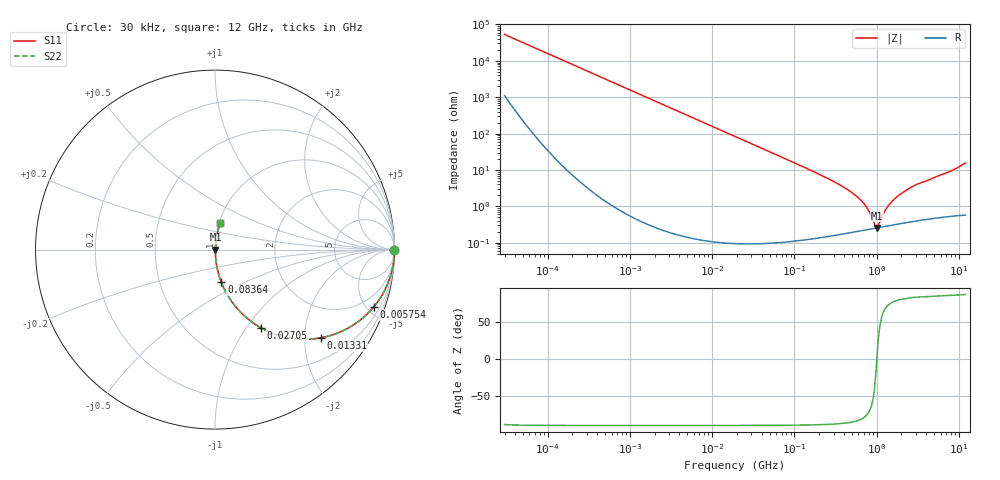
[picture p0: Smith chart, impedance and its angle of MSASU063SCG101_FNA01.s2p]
! MSASU063SCG101_FNA01  S-PARAMETER MODEL  ( General Type )
! Model Generated by TAIYO YUDEN Corporation (http://www.ty-top.com)
! Version 1.0
! TAIYO YUDEN Control No. 130520
! Copyright(c) 2013 TAIYO YUDEN CO.,LTD. All Rights Reserved.
! Product Description (link to TY-COMPAS)
! https://ds.yuden.co.jp/TYCOMPAS/or/detail?pn=MSASU063SCG101JFNA01&u=M
! Products Name : Multilayer Ceramic Capacitors
! Characteristics :
!  Capacitance : 100 pF , Rated Voltage : 50V , TCC : CG / C0G
!  Case Size : 0.6 x 0.3 / 0.024 x 0.012 [mm/inch] , Thickness : 0.3 / 0.012 [mm/inch]
!  (Conditions: Temperature = 25 degC , DC Bias Current/Voltage = 0A / 0V)
! External Node Assignments :
!  1  o---| |---o  2
! GND o---------o GND
! Frequency Range : 0.03MHz  -  12000MHz  [ 401 STEP ]
# MHz S RI R 50
! Freq[MHz].  S11 Real  S11 Imag  S21 Real  S21 Imag  S12 Real  S12 Imag  S22 Real  S22 Imag
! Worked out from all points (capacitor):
!   401 points, 30 kHz to 12 GHz, reference 50 ohm
!   read as one part in series: C = 99.9 pF near 32 kHz
!   lowest |Z| = 256 mohm at 1.002 GHz (marker M1)
!   series resonance near 1.004 GHz, so ESL is about 250 pH
!   S11 on the Smith chart (normalised r, x): 30 kHz: open; 5.754 MHz: 1.00, -5.54; 13.31 MHz: 1.00, -2.39; 27.05 MHz: 1.00, -1.18; 83.64 MHz: 1.00, -0.38; 12 GHz: 1.01, +0.31
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0.03  1 -0.00188  4.27e-05 0.00188  4.27e-05 0.00188  1 -0.00188
0.260295  0.9997 -0.0163  0.000279 0.0163  0.000279 0.0163  0.9997 -0.0163
2.258455  0.9802 -0.139  0.0198 0.139  0.0198 0.139  0.9802 -0.139
5.753879  0.8844 -0.3195  0.1156 0.3195  0.1156 0.3195  0.8844 -0.3195
13.30744  0.5887 -0.4917  0.4113 0.4917  0.4113 0.4917  0.5887 -0.4917
18.97367  0.4133 -0.4919  0.5867 0.4919  0.5867 0.4919  0.4133 -0.4919
27.05253  0.2574 -0.4364  0.7426 0.4364  0.7426 0.4364  0.2574 -0.4364
45.32004  0.1102 -0.3118  0.8898 0.3118  0.8898 0.3118  0.1102 -0.3118
83.63502  0.0355 -0.1822  0.9645 0.1822  0.9645 0.1822  0.0355 -0.1822
164.6252  0.01 -0.0931  0.99 0.0931  0.99 0.0931  0.01 -0.0931
356.9603  0.00319 -0.0388  0.9968 0.0388  0.9968 0.0388  0.00319 -0.0388
560.6502  0.00239 -0.0195  0.9976 0.0195  0.9976 0.0195  0.00239 -0.0195
749.4426  0.00235 -0.00942  0.9976 0.00942  0.9976 0.00942  0.00235 -0.00942
939.2353  0.00249 -0.00217  0.9975 0.00217  0.9975 0.00217  0.00249 -0.00217
1001.808  0.00255 -8.18e-05  0.9974 8.18e-05  0.9974 8.18e-05  0.00255 -8.18e-05
1068.55  0.00263 0.00196  0.9974 -0.00196  0.9974 -0.00196  0.00263 0.00196
1255.512  0.00285 0.00682  0.9972 -0.00682  0.9972 -0.00682  0.00285 0.00682
1428.372  0.00307 0.0109  0.9969 -0.0109  0.9969 -0.0109  0.00307 0.0109
1848.769  0.00366 0.0197  0.9963 -0.0197  0.9963 -0.0197  0.00366 0.0197
2811.574  0.00513 0.0359  0.9949 -0.0359  0.9949 -0.0359  0.00513 0.0359
7890.678  0.0136 0.0906  0.9864 -0.0906  0.9864 -0.0906  0.0136 0.0906
12000  0.0291 0.1507  0.9709 -0.1507  0.9709 -0.1507  0.0291 0.1507
